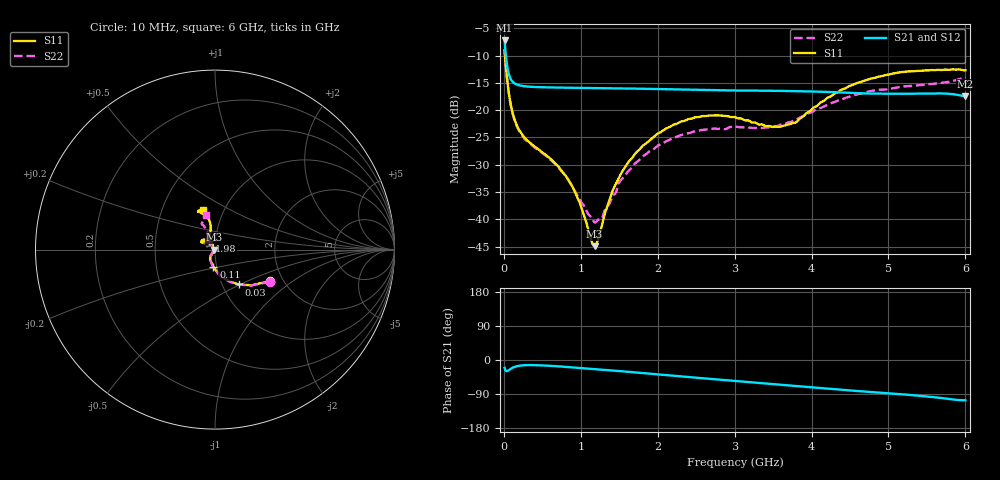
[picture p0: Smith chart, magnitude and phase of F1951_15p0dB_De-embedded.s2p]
! Integrated Device Technology
! Corporate Headquarters
! 6024 Silver Creek Valley Road
! San Jose, CA 95138  USA
! Phone:  1-408-284-8200
! Toll Free:  1-800-223-1366
! Webpage:  http://www.idt.com/
! Timing and RF Division
! 515 Groton Road, Suite 102
! Westford, MA 01886-6024
! Device:  F1951
! Description: 6-bit 0.5 dB Digital Step Attenuator
! Frequency:  100.0 -  4000.00 MHz
! Package:  4x4 mm Thin QFN Plastic Package: 24 pin
! Ports:  2 RF, 6 DC
!  Pin  1  = NC
!  Pin  2  = RF1  =  Port 1
!  Pin  3  = GND
!  Pin  4  = NC
!  Pin  5  = Serial Data Out (SDO)
!  Pin  6  = NC
!  Pin  7  = Reset Bar ( RSTb)
!  Pin  8  = Clock (CLK)
!  Pin  9  = Chip Select Bar (CSb)
!  Pin 10  = NC
!  Pin 11  = Serial Data In (SDI)
!  Pin 12  = NC
!  Pin 13  = NC
!  Pin 14  = VDD
!  Pin 15  = NC
!  Pin 16  = GND
!  Pin 17  = RF2  =  Port 2
!  Pin 18  = NC
!  Pin 19  = GND
!  Pin 20  = GND
!  Pin 21  = GND
!  Pin 22  = GND
!  Pin 23  = GND
!  Pin 24  = GND
! State:  30
! Atten State:  15.0 dB
! Voltage:  +3.30 Volts
! Current:  0.474 mA
! Data:  The device was measured on a F195X evaluation board which has
!  individual transmission lines to the RF pins.  Data was collected
!  de-embedded using a Automatic Fixture Removal [AFR] (Keysight Technologies).
!  The reference plane is the edge of the package pin.
! Misc:  Lot Code  1225BCA
!  Action Tracker AT0399
! Date Measured:  2018-09-13
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# GHz S dB R 50
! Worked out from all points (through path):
!   600 points, 10 MHz to 6 GHz, reference 50 ohm
!   highest |S21| = -7.23 dB at 10 MHz (marker M1); lowest = -17.4 dB at 6 GHz (marker M2)
!   group delay of S21, straight-line fit = 44.9 ps
!   lowest |S11| = -44.9 dB at 1.18 GHz (marker M3), VSWR 1.01, Z = 49.4 + j0.041 ohm
!   |S11| at or under -10 dB: 15.12 MHz to end of sweep
!   |S22| runs from -40.6 to -9.0 dB; largest |S21 - S12| = 0.00032
!   S11 on the Smith chart (normalised r, x): 10 MHz: 1.72, -0.69; 30 MHz: 1.20, -0.49; 110 MHz: 0.97, -0.19; 1.98 GHz: 0.93, +0.09; 6 GHz: 0.80, +0.38
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0.01  -9.00 -29.6  -7.23 -20.5  -7.23 -20.5  -8.98 -30.0
0.03  -12.56 -55.6  -10.51 -29.4  -10.50 -29.5  -12.63 -56.4
0.06  -16.37 -76.7  -13.16 -27.4  -13.16 -27.4  -16.50 -77.7
0.11  -20.31 -95.1  -14.73 -20.6  -14.74 -20.6  -20.40 -96.3
0.26  -24.85 -117.4  -15.60 -14.0  -15.60 -13.9  -25.09 -119.5
0.72  -30.54 -121.8  -15.87 -16.9  -15.87 -16.9  -30.71 -129.2
0.89  -33.98 -121.5  -15.92 -19.4  -15.91 -19.4  -34.01 -131.2
1.01  -37.93 -125.8  -15.95 -21.2  -15.95 -21.2  -36.92 -136.6
1.18  -44.92 175.8  -15.97 -23.9  -15.97 -23.9  -40.56 -170.7
1.27  -41.43 130.6  -15.98 -25.4  -15.98 -25.3  -39.95 162.2
1.39  -35.74 115.0  -16.00 -27.4  -16.00 -27.4  -36.59 139.4
1.52  -31.70 113.2  -16.03 -29.5  -16.03 -29.5  -32.86 130.8
1.72  -27.77 116.5  -16.06 -33.1  -16.06 -33.1  -29.61 128.4
1.98  -24.51 124.0  -16.13 -37.6  -16.13 -37.6  -26.76 131.6
2.01  -24.23 125.3  -16.14 -38.2  -16.14 -38.1  -26.44 132.7
2.49  -21.29 139.8  -16.26 -46.5  -16.26 -46.5  -23.88 142.4
3.01  -21.31 150.7  -16.39 -55.4  -16.39 -55.3  -23.03 146.9
3.59  -23.05 129.2  -16.47 -65.2  -16.47 -65.2  -22.70 128.3
4.01  -19.76 104.2  -16.58 -72.4  -16.59 -72.4  -20.31 115.7
4.49  -15.58 101.1  -16.82 -80.3  -16.82 -80.3  -17.53 114.3
5.01  -13.47 109.4  -17.00 -87.8  -17.00 -87.8  -16.18 117.1
6  -12.71 106.3  -17.45 -106.3  -17.45 -106.3  -14.00 105.2
